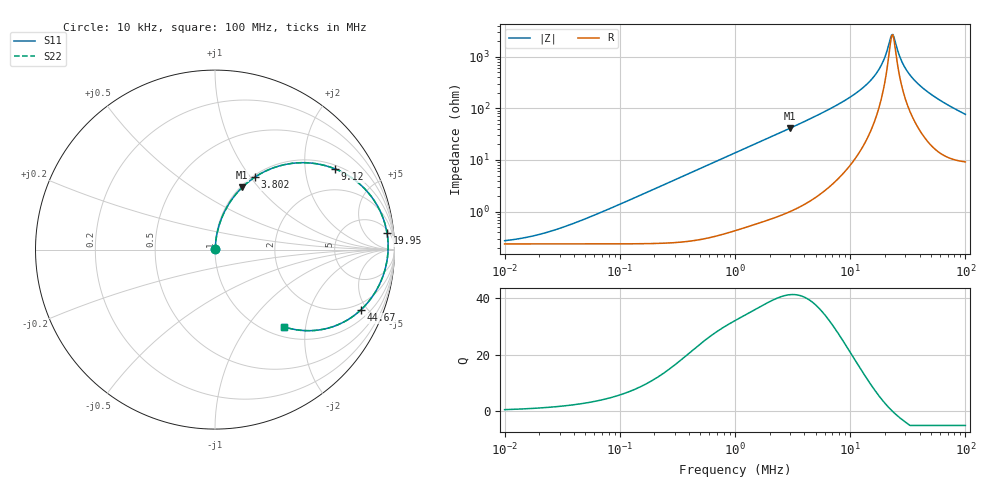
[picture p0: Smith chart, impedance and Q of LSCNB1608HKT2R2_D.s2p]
! LSCNB1608HKT2R2_D  S-PARAMETER MODEL  ( Standard Model )
! Model Generated by TAIYO YUDEN Corporation (http://www.ty-top.com)
! Version 1.0
! TAIYO YUDEN Control No. 200410
! Copyright(c) 2020 TAIYO YUDEN CO.,LTD. All Rights Reserved.
! Product Description (link to TY-COMPAS)
! https://ds.yuden.co.jp/TYCOMPAS/or/detail?pn=LSCNB1608HKT2R2MD&u=M
! Products Name : Inductors
! Characteristics :
!  Inductance : 2.2 [uH] , SRF(min) : - [Hz] , DC Resistance(max) : 292 [mOhm]
!  Rated Current : Saturation  1.5 [A] (dL = 30 [%]), Temp Rise  1.2 [A] (dT = 40 [degC])
!  Case Size : 1.6 x 0.8 / 0.063 x 0.031 [mm/inch] , Thickness : 0.8 / 0.031 [mm/inch]
!  (Conditions: Temperature = 25 [degC] , DC Bias Current = 0 [A])
! External Node Assignments :
!  1  o---GGG---o  2
! GND o---------o GND
! Frequency Range : 10kHz  -  100MHz  [ 402 STEP ]
# MHz S RI R 50
! Freq[MHz].  S11 Real  S11 Imag  S21 Real  S21 Imag  S12 Real  S12 Imag  S22 Real  S22 Imag
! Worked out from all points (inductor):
!   401 points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, 10 kHz to 100 MHz, reference 50 ohm
!   read as one part in series: L = 2.17 uH near 52.48 kHz
!   highest Q = 41.1 at 3.02 MHz (marker M1), where L = 2.18 uH
!   self-resonance near 22.91 MHz
!   S11 on the Smith chart (normalised r, x): 10 kHz: 1.00, +0.00; 3.802 MHz: 1.03, +1.05; 9.12 MHz: 1.12, +2.89; 19.95 MHz: 7, +18; 44.67 MHz: 1.53, -4.52; 100 MHz: 1.18, -1.52
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0.01  0.00237 0.00136  0.9976 -0.00136  0.9976 -0.00136  0.00237 0.00136
0.020893  0.00237 0.00284  0.9976 -0.00284  0.9976 -0.00284  0.00237 0.00284
0.046774  0.00241 0.00636  0.9976 -0.00636  0.9976 -0.00636  0.00241 0.00636
0.218776  0.00331 0.0298  0.9967 -0.0298  0.9967 -0.0298  0.00331 0.0298
1  0.0223 0.1327  0.9777 -0.1327  0.9777 -0.1327  0.0223 0.1327
3.019952  0.1519 0.347  0.8481 -0.347  0.8481 -0.347  0.1519 0.347
3.801894  0.2217 0.4033  0.7783 -0.4033  0.7783 -0.4033  0.2217 0.4033
4.677351  0.3047 0.4475  0.6953 -0.4475  0.6953 -0.4475  0.3047 0.4475
6.606934  0.4825 0.4843  0.5175 -0.4843  0.5175 -0.4843  0.4825 0.4843
9.120108  0.6696 0.4495  0.3304 -0.4495  0.3304 -0.4495  0.6696 0.4495
14.79108  0.8954 0.26  0.1046 -0.26  0.1046 -0.26  0.8954 0.26
17.37801  0.938 0.1714  0.062 -0.1714  0.062 -0.1714  0.938 0.1714
19.95262  0.9587 0.091  0.0413 -0.091  0.0413 -0.091  0.9587 0.091
21.87762  0.9643 0.0366  0.0357 -0.0366  0.0357 -0.0366  0.9643 0.0366
23.44229  0.9643 -0.00398  0.0357 0.00398  0.0357 0.00398  0.9643 -0.00398
24.54709  0.9624 -0.0308  0.0376 0.0308  0.0376 0.0308  0.9624 -0.0308
27.54229  0.9511 -0.0966  0.0489 0.0966  0.0489 0.0966  0.9511 -0.0966
30.19952  0.9358 -0.1474  0.0642 0.1474  0.0642 0.1474  0.9358 -0.1474
35.48134  0.8962 -0.2316  0.1038 0.2316  0.1038 0.2316  0.8962 -0.2316
44.66836  0.8112 -0.3373  0.1888 0.3373  0.1888 0.3373  0.8112 -0.3373
66.06934  0.6044 -0.4435  0.3956 0.4435  0.3956 0.4435  0.6044 -0.4435
100  0.3821 -0.4293  0.6179 0.4293  0.6179 0.4293  0.3821 -0.4293
